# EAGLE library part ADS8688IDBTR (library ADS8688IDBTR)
Octal Channel Single ADC SAR 500ksps 16-bit Serial 38-Pin TSSOP T/R Source: Datasheet
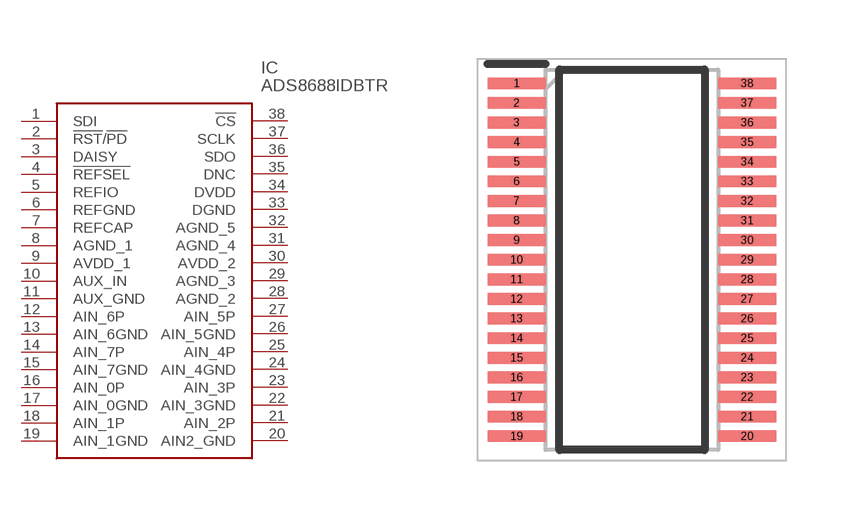
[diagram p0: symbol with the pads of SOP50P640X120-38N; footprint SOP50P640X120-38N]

Designator prefix IC

## ADS8688IDBTR (Description: Octal Channel Single ADC SAR 500ksps 16-bit Serial 38-Pin TSSOP T/R; Height: 1.2mm; Manufacturer_Name: Texas Instruments; Manufacturer_Part_Number: ADS8688IDBTR; Mouser_Part_Number: 595-ADS8688IDBTR; Mouser_Price-Stock: https://www.mouser.co.uk/ProductDetail/Texas-Instruments/ADS8688IDBTR?qs=bZA2O%252B%252B1GJuPFEagMJIgMw%3D%3D)  [SOP50P640X120-38N]
1  SDI
2  !RST!/!PD
3  DAISY
4  !REFSEL
5  REFIO
6  REFGND
7  REFCAP
8  AGND_1
9  AVDD_1
10  AUX_IN
11  AUX_GND
12  AIN_6P
13  AIN_6GND
14  AIN_7P
15  AIN_7GND
16  AIN_0P
17  AIN_0GND
18  AIN_1P
19  AIN_1GND
20  AIN2_GND
21  AIN_2P
22  AIN_3GND
23  AIN_3P
24  AIN_4GND
25  AIN_4P
26  AIN_5GND
27  AIN_5P
28  AGND_2
29  AGND_3
30  AVDD_2
31  AGND_4
32  AGND_5
33  DGND
34  DVDD
35  DNC
36  SDO
37  SCLK
38  !CS

## Footprint SOP50P640X120-38N (pad centres in mm)
DBT0038A
smd 1.475 x 0.3: 1 -2.938,4.5; 2 -2.938,4; 3 -2.938,3.5; 4 -2.938,3; 5 -2.938,2.5; 6 -2.938,2; 7 -2.938,1.5; 8 -2.938,1; 9 -2.938,0.5; 10 -2.938,0; 11 -2.938,-0.5; 12 -2.938,-1; 13 -2.938,-1.5; 14 -2.938,-2; 15 -2.938,-2.5; 16 -2.938,-3; 17 -2.938,-3.5; 18 -2.938,-4; 19 -2.938,-4.5; 20 2.938,-4.5; 21 2.938,-4; 22 2.938,-3.5; 23 2.938,-3; 24 2.938,-2.5; 25 2.938,-2; 26 2.938,-1.5; 27 2.938,-1; 28 2.938,-0.5; 29 2.938,0; 30 2.938,0.5; 31 2.938,1; 32 2.938,1.5; 33 2.938,2; 34 2.938,2.5; 35 2.938,3; 36 2.938,3.5; 37 2.938,4; 38 2.938,4.5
